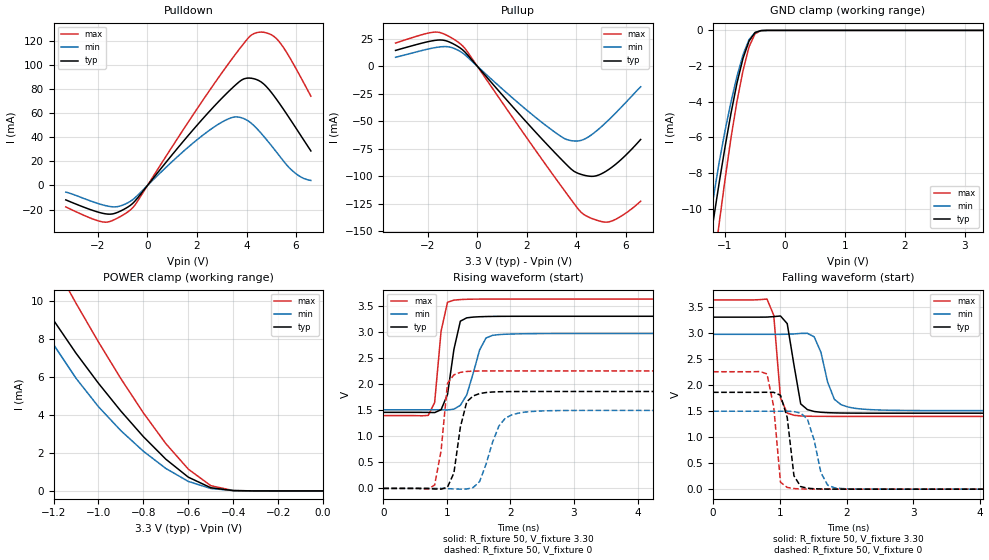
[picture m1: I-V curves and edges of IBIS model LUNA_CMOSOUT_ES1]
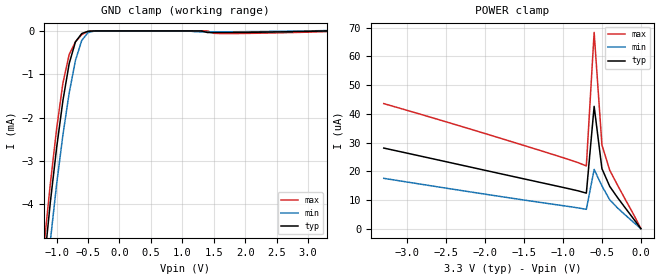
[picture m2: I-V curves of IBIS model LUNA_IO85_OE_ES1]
[IBIS Ver]   3.2
[Comment Char]   |_char
[File name]   sg-8018cx_33v_b.ibs
[File Rev]   1.0
[Date]   2017/01/25 2:19:36
[Source]
[Notes]
[Disclaimer]
This information is for modeling purposes only, and is not guaranteed.
Property of SEIKO EPSON Corp.,
unauthorized reproduction and/or distribution is strictly prohibited.
[Copyright]
Copyright 2017, SEIKO EPSON Corp.
[Component]   SG-8018CA
Si_location Pin
Timing_location Pin
[Manufacturer]   SEIKO EPSON Corp.
| 7050 PKG
| 7050 PKG
[Package]
R_pkg   224m   NA   NA
L_pkg   5.5n   NA   NA
C_pkg   0.144p   NA   NA
[Pin] signal_name   model_name
1   OE   LUNA_IO85_OE_ES1
2   VSS   GND
3   OUT   LUNA_CMOSOUT_ES1
4   VDD   POWER
[Component]   SG-8018CB
Si_location Pin
Timing_location Pin
[Manufacturer]   SEIKO EPSON Corp.
| 5032 PKG
| 5032 PKG
[Package]
R_pkg   200m   NA   NA
L_pkg   2.16n   NA   NA
C_pkg   1.23p   NA   NA
[Pin] signal_name   model_name
1   OE   LUNA_IO85_OE_ES1
2   VSS   GND
3   OUT   LUNA_CMOSOUT_ES1
4   VDD   POWER
[Component]   SG-8018CE
Si_location Pin
Timing_location Pin
[Manufacturer]   SEIKO EPSON Corp.
| 3225 PKG
| 3225 PKG
[Package]
R_pkg   177m   NA   NA
L_pkg   4.5n   NA   NA
C_pkg   0.64p   NA   NA
[Pin] signal_name   model_name
1   OE   LUNA_IO85_OE_ES1
2   VSS   GND
3   OUT   LUNA_CMOSOUT_ES1
4   VDD   POWER
[Component]   SG-8018CG
Si_location Pin
Timing_location Pin
[Manufacturer]   SEIKO EPSON Corp.
| 2520 PKG
| 2520 PKG
[Package]
R_pkg   238m   NA   NA
L_pkg   2.1n   NA   NA
C_pkg   0.38p   NA   NA
[Pin] signal_name   model_name
1   OE   LUNA_IO85_OE_ES1
2   VSS   GND
3   OUT   LUNA_CMOSOUT_ES1
4   VDD   POWER
| Models and submodels in the file (2): LUNA_CMOSOUT_ES1 (3-state), LUNA_IO85_OE_ES1 (Input)
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[Model]   LUNA_CMOSOUT_ES1
Model_type 3-state
Enable Active-High
Polarity Non-Inverting
Vmeas=1.65
C_comp   2.5p   2.0p   3.0p
[Temperature Range] 25   105   -40
[Voltage Range]   3.30   2.97   3.63
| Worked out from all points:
|   slope of the pulldown table from 0 to 0.495 V, typ, clamps not added: 38.8 ohm
|   slope of the pullup table from 0 to 0.495 V, typ, clamps not added: 38.4 ohm
|   GND clamp passes 1 mA (typ) near -0.64 V on its own axis
|   POWER clamp passes 1 mA (typ) near -0.63 V on its own axis
|   falling waveform, R_fixture 50, V_fixture 3.30: 20-80 % time 145ps typ, 196ps min, 85.4ps max; typ from 3.3 V to 1.46 V
|   falling waveform, R_fixture 50, V_fixture 0: 20-80 % time 117ps typ, 172ps min, 115ps max; typ from 1.86 V to 0 V
|   rising waveform, R_fixture 50, V_fixture 3.30: 20-80 % time 148ps typ, 211ps min, 118ps max; typ from 1.46 V to 3.3 V
|   rising waveform, R_fixture 50, V_fixture 0: 20-80 % time 157ps typ, 253ps min, 126ps max; typ from 0 V to 1.86 V
[Pullup]
-3.3V     14.33mA    8.077mA    21.05mA
-1.6V     23.72mA    17.26mA    30.95mA
-1.1V     21.71mA    17.34mA    26.52mA
-600mV    15.01mA    12.11mA    18.66mA
2.4V      -61.05mA   -47.37mA   -77.98mA
3.4V      -84.85mA   -64.2mA    -109.4mA
3.8V      -93.77mA   -67.77mA   -121.6mA
4.3V      -99.11mA   -66.66mA   -134.8mA
4.7V      -100.2mA   -60.99mA   -139.2mA
5.2V      -95.57mA   -51.2mA    -141.9mA
5.8V      -85.15mA   -37.72mA   -136.6mA
6.6V      -66.67mA   -18.75mA   -122.8mA
[Pulldown]
-3.3V     -11.97mA   -5.469mA   -17.78mA
-1.7V     -23.51mA   -16.69mA   -30.44mA
-1.2V     -22.23mA   -17.52mA   -26.92mA
-700mV    -16.6mA    -13.24mA   -20.43mA
1.5V      37.88mA    29.13mA    47.95mA
2.9V      70.1mA     51.21mA    90.31mA
3.6V      84.07mA    56.84mA    110mA
4.3V      88.44mA    49.59mA    125.9mA
4.8V      82mA       38.16mA    126.5mA
5.3V      68.83mA    25.32mA    119.7mA
6V        47.43mA    9.721mA    96.77mA
6.6V      28.59mA    4.146mA    73.95mA
[GND Clamp]
-3.3V     -86.74mA   -76.76mA   -101.8mA
-1.3V     -13.11mA   -11.85mA   -16.24mA
-1.2V     -10.77mA   -9.503mA   -13.52mA
-1.1V     -8.591mA   -7.44mA    -10.88mA
-1V       -6.541mA   -5.623mA   -8.358mA
-900mV    -4.635mA   -4.001mA   -6.009mA
-800mV    -2.939mA   -2.563mA   -3.961mA
-700mV    -1.565mA   -1.365mA   -2.263mA
-600mV    -601.2uA   -521.6uA   -925.2uA
-500mV    -121.4uA   -116.4uA   -188.8uA
-300mV    -500.8nA   -1.29uA    -313.6nA
3.3V      193.1pA    4.095uA    131.4pA
[POWER Clamp]
-3.3V     73.68mA    63.39mA    89.04mA
-1.4V     13.2mA     11.93mA    16.56mA
-1.3V     10.93mA    9.714mA    14.21mA
-1.2V     8.97mA     7.69mA     11.99mA
-1.1V     7.236mA    5.92mA     9.861mA
-1V       5.655mA    4.424mA    7.824mA
-900mV    4.191mA    3.162mA    5.894mA
-700mV    1.665mA    1.179mA    2.483mA
-600mV    721.7uA    498.7uA    1.143mA
-500mV    167.2uA    126.9uA    275.1uA
-400mV    16.41uA    18.75uA    19.76uA
0V        193.1pA    1.068nA    160pA
[Falling Waveform]
R_fixture=50
V_fixture=3.30
V_fixture_min=2.97
V_fixture_max=3.63
0s        3.3V       2.97V      3.63V
808.1ps   3.301V     2.97V      3.647V
909.1ps   3.311V     2.97V      3.337V
1.01ns    3.322V     2.97V      1.75V
1.111ns   3.176V     2.973V     1.46V
1.212ns   2.384V     2.978V     1.418V
1.414ns   1.526V     2.99V      1.4V
1.818ns   1.463V     1.723V     1.396V
2.121ns   1.459V     1.552V     1.396V
10ns      1.458V     1.507V     1.396V
[Falling Waveform]
R_fixture=50
V_fixture=0
V_fixture_min=0
V_fixture_max=0
0s        1.858V     1.495V     2.253V
808.1ps   1.859V     1.495V     2.211V
909.1ps   1.857V     1.495V     1.579V
1.01ns    1.801V     1.495V     134.5mV
1.111ns   1.375V     1.496V     32.71mV
1.212ns   256.7mV    1.489V     12mV
1.313ns   49.34mV    1.459V     4.672mV
1.616ns   3.616mV    315.2mV    332.4uV
1.818ns   943.9uV    27.32mV    70.2uV
10ns      -2.857uV   0V         -3.951uV
[Rising Waveform]
R_fixture=50
V_fixture=3.30
V_fixture_min=2.97
V_fixture_max=3.63
0s        1.458V     1.507V     1.396V
707.1ps   1.457V     1.507V     1.399V
808.1ps   1.453V     1.507V     1.647V
909.1ps   1.508V     1.507V     3.013V
1.01ns    1.801V     1.504V     3.568V
1.111ns   2.665V     1.519V     3.609V
1.212ns   3.206V     1.593V     3.621V
1.515ns   3.291V     2.654V     3.629V
1.717ns   3.297V     2.934V     3.63V
10ns      3.3V       2.97V      3.63V
[Rising Waveform]
R_fixture=50
V_fixture=0
V_fixture_min=0
V_fixture_max=0
0s        0V         0V         0V
808.1ps   -11.1mV    34.24uV    65.82mV
909.1ps   -14.54mV   241.3uV    722mV
1.01ns    25.3mV     -4.285mV   2.015V
1.111ns   295.8mV    -10.83mV   2.178V
1.212ns   1.173V     -13.96mV   2.225V
1.414ns   1.773V     17.07mV    2.248V
1.818ns   1.853V     1.195V     2.253V
2.222ns   1.858V     1.462V     2.253V
10ns      1.858V     1.495V     2.253V
[Ramp]
R_load=50
dV/dt_r   1.115E+0/1.512E-10   8.970E-1/2.496E-10   1.352E+0/1.112E-10
dV/dt_f   1.105E+0/1.365E-10   8.778E-1/1.770E-10   1.341E+0/7.841E-11
|[End   LUNA_CMOSOUT_ES1
[Model]   LUNA_IO85_OE_ES1
Model_type Input
Enable Active-Low
Polarity Non-Inverting
Vinh=2.55
Vinl=0.89
C_comp   2.5p   2.0p   3.0p
[Temperature Range] 25   105   -40
[Voltage Range]   3.30   2.97   3.63
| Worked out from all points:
|   GND clamp passes 1 mA (typ) near -0.83 V on its own axis
[GND Clamp]
-3.3V     -49.97mA   -47.74mA   -53.94mA
-1.2V     -5.408mA   -6.351mA   -4.953mA
-1.1V     -3.959mA   -4.854mA   -3.533mA
-1V       -2.702mA   -3.543mA   -2.264mA
-900mV    -1.612mA   -2.406mA   -1.207mA
-800mV    -755.8uA   -1.435mA   -544.3uA
-700mV    -251.9uA   -680.1uA   -254.3uA
-600mV    -60.6uA    -218.5uA   -85.08uA
-500mV    -8.506uA   -39.85uA   -10.99uA
-400mV    -1.005uA   -4.241uA   -1.145uA
1.7V      -37.51uA   -20.16uA   -61.79uA
3.3V      135.9pA    8.008uA    -15.73uA
[POWER Clamp]
-3.3V     28.08uA    17.53uA    43.56uA
-1.6V     17.94uA    10.38uA    29.81uA
-900mV    13.77uA    7.613uA    23.86uA
-700mV    12.37uA    6.737uA    21.84uA
-600mV    42.62uA    20.63uA    68.38uA
-500mV    20.91uA    14.89uA    29.15uA
-400mV    14.72uA    10.06uA    20.36uA
-300mV    10.84uA    7.224uA    15.17uA
-100mV    3.62uA     2.354uA    5.264uA
0V        135.7pA    303.7pA    135.4pA
